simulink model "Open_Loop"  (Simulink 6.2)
settings: Solver=ode45  StartTime=0.0  StopTime=10  FixedStep=0.04  RelTol=1e-3
undefined symbols (not defined in the file or in its folder): Ac, As, At, Av, Bc, Bs, Bt, Bv, Cc, Cs, Ct, Cv, Dc, Ds, Dt, Dv

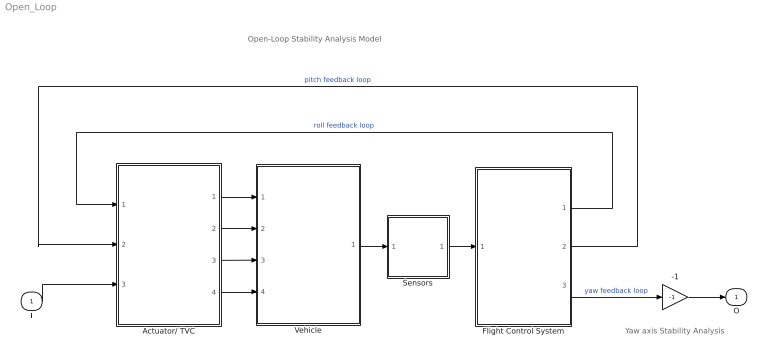
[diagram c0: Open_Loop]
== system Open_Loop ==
  note: Open-Loop Stability Analysis Model
  note: Yaw axis Stability Analysis
  I : Inport  Port=1  LatchInput=off
  -1 : Gain  Gain=-1
  Actuator/ TVC : Subsystem
  Flight Control System : Subsystem
  Sensors : Subsystem
  Vehicle : Subsystem
  O : Outport
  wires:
  -1/1 -> O/1
  Vehicle/1(meas) -> Sensors/1(meas)
  Sensors/1(sens) -> Flight Control System/1(measur)
  Actuator/ TVC/1(DY) -> Vehicle/1(DY)
  Actuator/ TVC/2(DY-dd) -> Vehicle/2(DY_dd)
  Actuator/ TVC/3(DZ) -> Vehicle/3(DZ)
  Actuator/ TVC/4(DZ-dd) -> Vehicle/4(DZ_dd)
  Flight Control System/1(DP-TVC) -> Actuator/ TVC/1(DP_tvc)  "roll feedback loop"
  I/1 -> Actuator/ TVC/3(DR_tvc)
  Flight Control System/3(DR-TVC) -> -1/1  "yaw feedback loop"
  Flight Control System/2(DQ-TVC) -> Actuator/ TVC/2(DQ_tvc)  "pitch feedback loop"

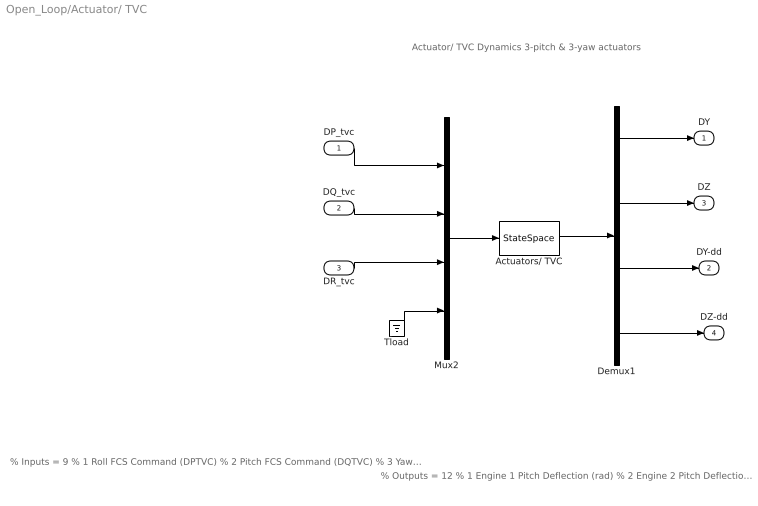
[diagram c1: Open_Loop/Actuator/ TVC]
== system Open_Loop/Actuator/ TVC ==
  note: Actuator/ TVC Dynamics 3-pitch & 3-yaw actuators
  note: % Inputs = 9 % 1 Roll FCS Command (DPTVC) % 2 Pitch FCS Command (DQTVC) % 3 Yaw FCS Command (DRTVC) % 4 Engine 1 Pitch Load-Torque TLY1 % 5 Engine 2 Pitch Load-Torque TLY2 % 6 Engine 3 Pitch Load-Torque TLY3 % 7 Engine 1 Yaw Load-Torque TLZ1 % 8 Engine 2 Yaw Load-Torque TLZ2 % 9 Engine 3 Yaw Load-Torque TLZ3
  note: % Outputs = 12 % 1 Engine 1 Pitch Deflection (rad) % 2 Engine 2 Pitch Deflection (rad) % 3 Engine 3 Pitch Deflection (rad) % 4 Engine 1 Yaw Deflection (rad) % 5 Engine 2 Yaw Deflection (rad) % 6 Engine 3 Yaw Deflection (rad) % 7 Engine 1 Pitch Accelerat (rad/sec^2) % 8 Engine 2 Pitch Accelerat (rad/sec^2) % 9 Engine 3 Pitch Accelerat (rad/sec^2) % 10 Engine 1 Yaw Accelerat (rad/sec^2) % 11 Engine 2 Yaw Accelerat (rad/sec^2) % 12 Engine 3 Yaw Accelerat (rad/sec^2)
  DP_tvc : Inport  Port=1  LatchInput=off
  DQ_tvc : Inport  Port=2  LatchInput=off
  DR_tvc : Inport  Port=3  LatchInput=off
  Actuators/ TVC : StateSpace  A=At  B=Bt  C=Ct  D=Dt
  Demux1 : Demux  Outputs=[3, 3, 3, 3]
  Mux2 : Mux  Inputs="[1, 1, 1,  6]"
  Tload : Ground
  DY : Outport
  DY-dd : Outport  Port=2
  DZ : Outport  Port=3
  DZ-dd : Outport  Port=4
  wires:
  Mux2/1 -> Actuators/ TVC/1
  Actuators/ TVC/1 -> Demux1/1
  Tload/1 -> Mux2/4
  DR_tvc/1 -> Mux2/3
  DQ_tvc/1 -> Mux2/2
  DP_tvc/1 -> Mux2/1
  Demux1/1 -> DY/1
  Demux1/2 -> DZ/1
  Demux1/4 -> DZ-dd/1
  Demux1/3 -> DY-dd/1

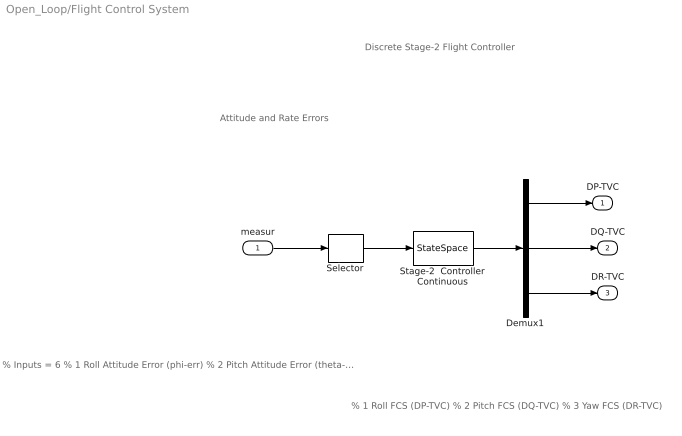
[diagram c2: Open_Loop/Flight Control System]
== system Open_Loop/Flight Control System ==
  note: Discrete Stage-2 Flight Controller
  note: Attitude and Rate Errors
  note: % Inputs = 6 % 1 Roll Attitude Error (phi-err) % 2 Pitch Attitude Error (theta-err) % 3 Yaw Attitude Error (psi-err) % 4 Roll Rate Error (p-err) % 5 Pitch Rate Error (q-err) % 6 Yaw Rate Error (r-err)
  note: % 1 Roll FCS (DP-TVC) % 2 Pitch FCS (DQ-TVC) % 3 Yaw FCS (DR-TVC)
  measur : Inport  Port=1  LatchInput=off
  Demux1 : Demux  Outputs=3
  Selector : Selector  Elements=[1 3 5 2 4 6]  InputPortWidth=6
  Stage-2  Controller Continuous : StateSpace  A=Ac  B=Bc  C=Cc  D=Dc
  DP-TVC : Outport
  DQ-TVC : Outport  Port=2
  DR-TVC : Outport  Port=3
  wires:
  Stage-2  Controller Continuous/1 -> Demux1/1
  Demux1/2 -> DQ-TVC/1
  Demux1/1 -> DP-TVC/1
  Demux1/3 -> DR-TVC/1
  measur/1 -> Selector/1
  Selector/1 -> Stage-2  Controller Continuous/1

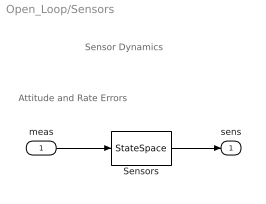
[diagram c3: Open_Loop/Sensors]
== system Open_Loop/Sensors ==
  note: Sensor Dynamics
  note: Attitude and Rate Errors
  meas : Inport  Port=1  LatchInput=off
  Sensors : StateSpace  A=As  B=Bs  C=Cs  D=Ds
  sens : Outport
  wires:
  meas/1 -> Sensors/1
  Sensors/1 -> sens/1

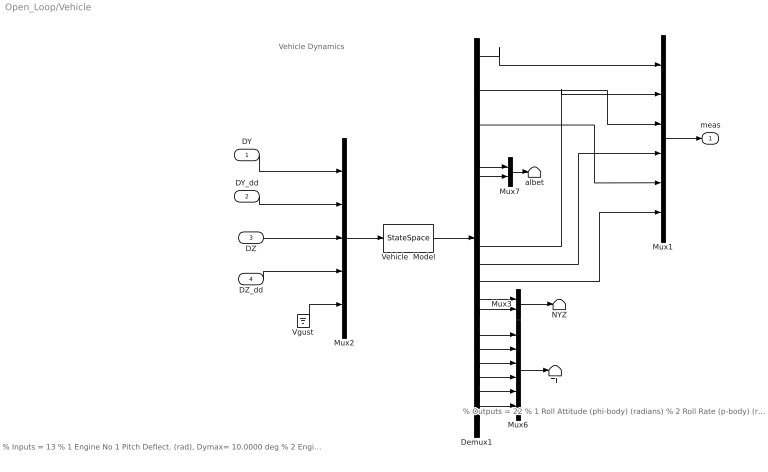
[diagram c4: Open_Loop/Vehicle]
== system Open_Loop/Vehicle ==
  note: Vehicle Dynamics
  note: % Inputs = 13 % 1 Engine No 1 Pitch Deflect. (rad), Dymax= 10.0000 deg % 2 Engine No 2 Pitch Deflect. (rad), Dymax= 10.0000 deg % 3 Engine No 3 Pitch Deflect. (rad), Dymax= 10.0000 deg % 4 Engine No 1 Pitch Acceleration (rad/sec^2) % 5 Engine No 2 Pitch Acceleration (rad/sec^2) % 6 Engine No 3 Pitch Acceleration (rad/sec^2) % 7 Engine No 1 Yaw Deflect. (rad), Dzmax= 10.0000 deg % 8 Engine No 2 Yaw Deflect. (rad), Dzmax= 10.0000 deg % 9 Engine No 3 Yaw Deflect. (rad), Dzmax= 10.0000 deg % 10 Engine No 1 Yaw Acceleration (rad/sec^2) % 11 Engine No 2 Yaw Acceleration (rad/sec^2) % 12 Engine No 3 Yaw Acceleration (rad/sec^2) % 13 Wind Gust Azim, Elev Angles=( 45.0 90.0) (deg)
  note: % Outputs = 22 % 1 Roll Attitude (phi-body) (radians) % 2 Roll Rate (p-body) (rad/sec) % 3 Pitch Attitude (thet-bdy) (radians) % 4 Pitch Rate (q-body) (rad/sec) % 5 Yaw Attitude (psi-body) (radians) % 6 Yaw Rate (r-body) (rad/sec) % 7 Angle of attack, alfa, (radians) % 8 Angle of sideslip, beta, (radian) % 9 Change in Altitude, delta-h, (feet) % 10 Forward Acceleration (V-dot) (ft/sec) % 11 Cross Range Velocity (Vcr) (ft/sec) % 12 Rate-Gyro # 1, Roll Rate (Body) (rad/sec) % 13 Rate-Gyro # 2, Pitch Rate (Body) (rad/sec) % 14 Rate-Gyro # 3, Yaw Rate (Body) (rad/sec) % 15 Accelerom # 1, (along Z), (ft/sec^2) Translat. Acceler % 16 Accelerom # 2, (along Y), (ft/sec^2) Translat. Acceler % 17 Ptch Load-Torque Tly for Engine: 1,(ft-lb) % 18 Ptch Load-Torque Tly for Engine: 2,(ft-lb) % 19 Ptch Load-Torque Tly for Engine: 3,(ft-lb) % 20 Yaw Load-Torque Tlz for Engine: 1,(ft-lb) % 21 Yaw Load-Torque Tlz for Engine: 2,(ft-lb) % 22 Yaw Load-Torque Tlz for Engine: 3,(ft-lb)
  DY : Inport  Port=1  LatchInput=off
  DY_dd : Inport  Port=2  LatchInput=off
  DZ : Inport  Port=3  LatchInput=off
  DZ_dd : Inport  Port=4  LatchInput=off
  Demux1 : Demux  Outputs=22
  Mux1 : Mux  Inputs=6
  Mux2 : Mux  Inputs=[3, 3, 3, 3, 1]
  Mux3 : Mux  Inputs=2
  Mux6 : Mux  Inputs=6
  Mux7 : Mux  Inputs=2
  NYZ : Terminator
  TL : Terminator
  Vehicle  Model : StateSpace  A=Av  B=Bv  C=Cv  D=Dv
  Vgust : Ground
  albet : Terminator
  meas : Outport
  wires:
  Mux7/1 -> albet/1
  Mux2/1 -> Vehicle  Model/1
  Vehicle  Model/1 -> Demux1/1
  Demux1/15 -> Mux3/1
  Demux1/16 -> Mux3/2
  Mux3/1 -> NYZ/1
  Demux1/22 -> Mux6/6
  Demux1/21 -> Mux6/5
  Demux1/20 -> Mux6/4
  Demux1/19 -> Mux6/3
  Demux1/18 -> Mux6/2
  Demux1/17 -> Mux6/1
  Mux6/1 -> TL/1
  Demux1/14 -> Mux1/6
  Demux1/13 -> Mux1/4
  Demux1/12 -> Mux1/2
  Demux1/7 -> Mux7/1
  Demux1/8 -> Mux7/2
  DY/1 -> Mux2/1
  DY_dd/1 -> Mux2/2
  DZ/1 -> Mux2/3
  Vgust/1 -> Mux2/5
  DZ_dd/1 -> Mux2/4
  Demux1/1 -> Mux1/1
  Demux1/3 -> Mux1/3
  Demux1/5 -> Mux1/5
  Mux1/1 -> meas/1
